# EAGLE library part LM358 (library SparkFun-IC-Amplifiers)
LM358 Jellybean op-amp Datasheet SparkFun Products Op-Amp (Thru-Hole) - LM358 (COM-09456)
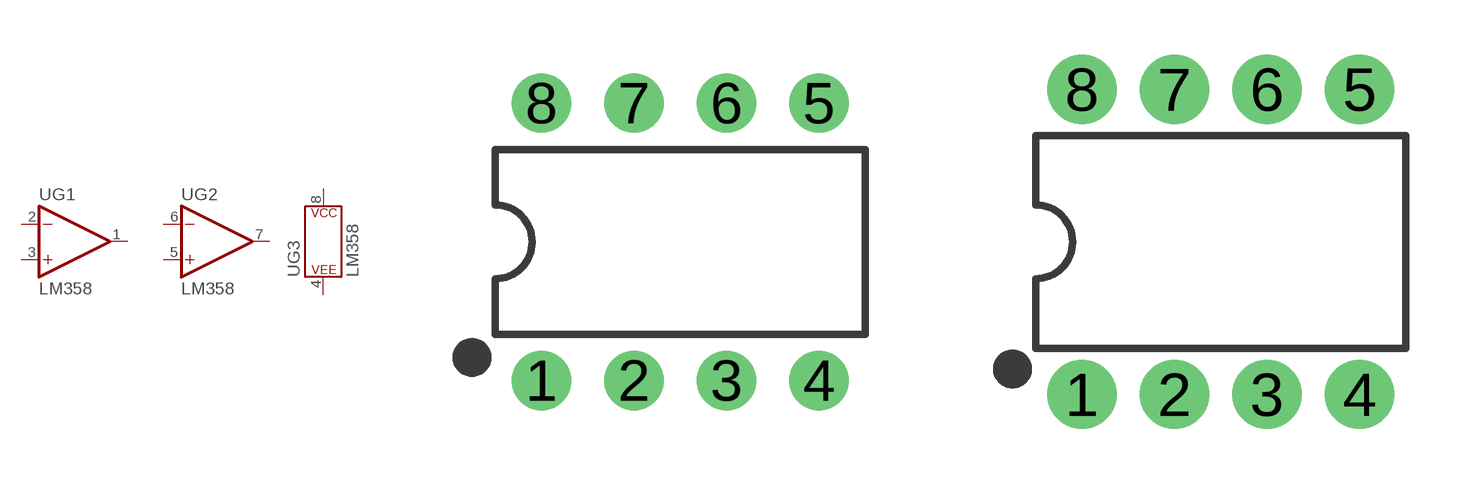
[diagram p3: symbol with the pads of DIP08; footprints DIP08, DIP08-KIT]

Designator prefix U; gates G1=OP-AMP G2=OP-AMP G3=POWER_CONSORT

## LM358 (PROD_ID: IC-09172; VALUE: LM358)  [DIP08]
1  G1:OUT  out
2  G1:-IN  in
3  G1:+IN  in
4  G3:P$V-
5  G2:+IN  in
6  G2:-IN  in
7  G2:OUT  out
8  G3:P$V+

## LM358KIT (PROD_ID: IC-09172; VALUE: LM358)  [DIP08-KIT]
Pads as for DIP08

## Footprint DIP08 (pad centres in mm)
Dual In Line Package
drill 0.813 pad 1.626: 1 -3.81,-3.81; 2 -1.27,-3.81; 3 1.27,-3.81; 4 3.81,-3.81; 5 3.81,3.81; 6 1.27,3.81; 7 -1.27,3.81; 8 -3.81,3.81

## Footprint DIP08-KIT (pad centres in mm)
drill 0.813 pad 1.905: 1 -3.81,-4.191; 2 -1.27,-4.191; 3 1.27,-4.191; 4 3.81,-4.191; 5 3.81,4.191; 6 1.27,4.191; 7 -1.27,4.191
drill 0.864 pad 1.905: 8 -3.81,4.191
